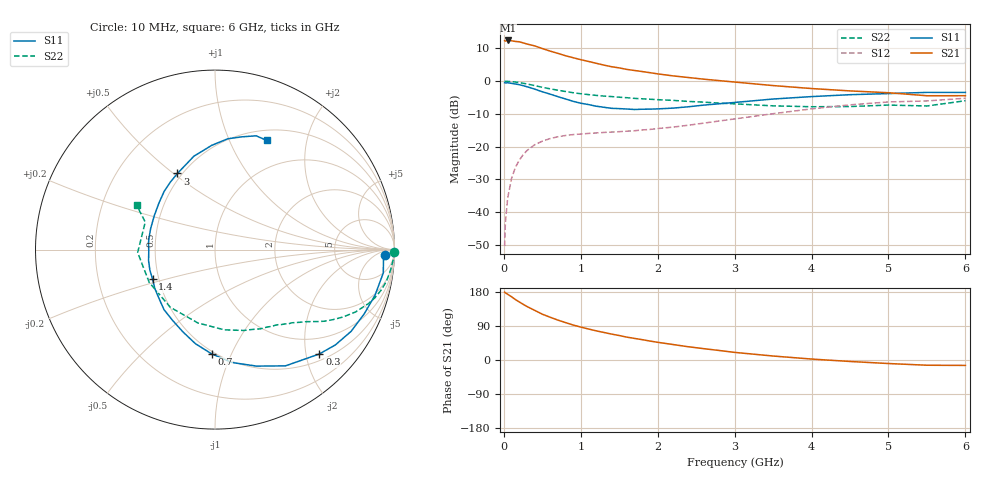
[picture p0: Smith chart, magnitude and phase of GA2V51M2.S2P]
! Infineon Technologies  Discrete & RF Semiconductors
! BF775
! Si NPN RF Bipolar Junction Transistor in SOT23
! VCE = 2.5 V  IC = 1.2 mA
! Common Emitter S-Parameters:  May  1996
# GHz  S  MA  R  50
!  f  S11  S21  S12  S22
! GHz  MAG  ANG  MAG  ANG  MAG  ANG  MAG  ANG
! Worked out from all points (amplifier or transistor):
!   36 points, 10 MHz to 6 GHz, reference 50 ohm
!   highest |S21| = 12.5 dB at 50 MHz (marker M1)
!   |S21| within 3 dB of that: start of sweep to 568.1 MHz
!   unconditionally stable (mu >= 1): 1.341 GHz to 4.4 GHz; 5.001 GHz to end of sweep
!   at 250 MHz: K = 0.22, MSG = 17.1 dB, |S12| = -22.5 dB
!   at 1.4 GHz: K = 1.03, MAG = 8.9 dB, |S12| = -15.6 dB
!   at 6 GHz: K = 1.03, MAG = -0.7 dB, |S12| = -5.2 dB
!   S11 on the Smith chart (normalised r, x): 10 MHz: 28, -16; 300 MHz: 0.63, -2.27; 700 MHz: 0.48, -0.84; 1.4 GHz: 0.46, -0.18; 3 GHz: 0.47, +0.52; 6 GHz: 0.62, +1.39
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0.01  0.9475 -1.7  4.163 179.0  0.003 89.5  0.9997 -0.7
0.02  0.9401 -3.1  4.097 177.2  0.0068 85.5  0.9946 -1.4
0.05  0.9466 -7.9  4.196 173.4  0.0164 84.9  0.9938 -3.5
0.1  0.9272 -15.9  4.154 166.9  0.0325 80.6  0.9836 -7.0
0.15  0.9053 -23.3  4.053 159.5  0.048 75.5  0.9714 -10.5
0.2  0.8846 -31.0  4.007 153.3  0.0617 70.8  0.9528 -13.7
0.3  0.8223 -45.0  3.702 141.2  0.0868 63.2  0.9072 -19.3
0.4  0.7574 -58.8  3.468 131.1  0.1065 56.4  0.8571 -23.9
0.5  0.689 -70.4  3.155 120.9  0.1209 50.7  0.8056 -27.8
0.6  0.6352 -81.7  2.888 113.0  0.1323 46.3  0.7644 -30.7
0.7  0.5809 -91.9  2.671 105.5  0.1411 42.7  0.7286 -33.2
0.9  0.4921 -111.3  2.286 92.4  0.1526 38.0  0.6664 -37.0
1.1  0.4393 -130.2  2.005 81.8  0.1589 35.5  0.6234 -40.5
1.4  0.3847 -154.8  1.664 68.4  0.1667 34.0  0.5818 -45.3
1.7  0.369 -179.1  1.457 56.9  0.1748 35.6  0.5456 -50.1
2.2  0.3875 150.9  1.205 40.8  0.1986 38.9  0.5087 -60.2
3  0.473 116.3  0.97 20.1  0.2648 40.9  0.4502 -83.3
3.5  0.5336 102.7  0.857 10.5  0.3183 38.3  0.4197 -103.2
4.5  0.6216 83.4  0.71 -3.9  0.4347 26.9  0.4095 -153.5
5  0.6463 76.5  0.666 -9.3  0.4815 19.1  0.4312 -177.8
5.5  0.6742 70.1  0.599 -13.8  0.4991 10.4  0.4177 158.5
6  0.673 64.6  0.6 -14.3  0.548 5.9  0.5024 150.4
